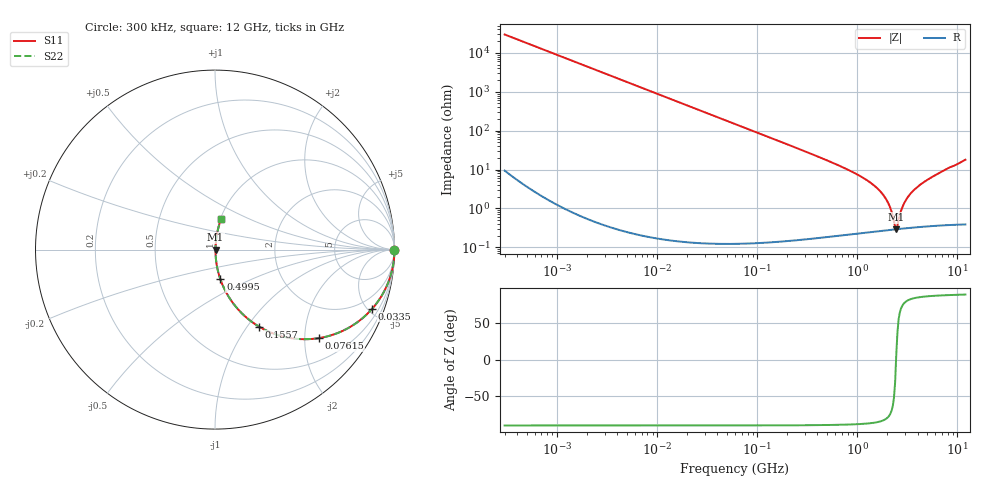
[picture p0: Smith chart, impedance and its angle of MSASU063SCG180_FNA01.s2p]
! MSASU063SCG180_FNA01  S-PARAMETER MODEL  ( Standard Model )
! Model Generated by TAIYO YUDEN Corporation (http://www.ty-top.com)
! Version 1.0
! TAIYO YUDEN Control No. 240819
! Copyright(c) 2024 TAIYO YUDEN CO.,LTD. All Rights Reserved.
! Product Description (link to TY-COMPAS)
! https://ds.yuden.co.jp/TYCOMPAS/or/detail?pn=MSASU063SCG180JFNA01&u=M
! Products Name : Multilayer Ceramic Capacitors
! Characteristics :
!  Capacitance : 18 [pF] , Rated Voltage : 50 [V] , TCC : CG / C0G
!  Case Size : 0.6 x 0.3 / 0.024 x 0.012 [mm/inch] , Thickness : 0.3 / 0.012 [mm/inch]
!  (Conditions: Temperature = 25 [degC] , DC Bias Voltage = 0 [V])
! External Node Assignments :
!  1  o---| |---o  2
! GND o---------o GND
! Frequency Range : 0.3MHz  -  12000MHz  [ 401 STEP ]
# MHZ S RI R 50
! Freq[MHz].  S11 Real  S11 Imag  S21 Real  S21 Imag  S12 Real  S12 Imag  S22 Real  S22 Imag
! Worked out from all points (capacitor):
!   401 points, 300 kHz to 12 GHz, reference 50 ohm
!   read as one part in series: C = 17.8 pF near 316.3 kHz
!   lowest |Z| = 293 mohm at 2.448 GHz (marker M1)
!   series resonance near 2.438 GHz, so ESL is about 240 pH
!   S11 on the Smith chart (normalised r, x): 300 kHz: open; 33.5 MHz: 1.00, -5.33; 76.15 MHz: 1.00, -2.34; 155.7 MHz: 1.00, -1.14; 499.5 MHz: 1.00, -0.34; 12 GHz: 1.01, +0.36
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0.3  1 -0.00336  1.24e-05 0.00336  1.24e-05 0.00336  1 -0.00336
1.769972  0.9996 -0.0198  0.000396 0.0198  0.000396 0.0198  0.9996 -0.0198
10.44266  0.9865 -0.1155  0.0135 0.1155  0.0135 0.1155  0.9865 -0.1155
33.49947  0.8763 -0.329  0.1237 0.329  0.1237 0.329  0.8763 -0.329
60  0.6882 -0.4628  0.3118 0.4628  0.3118 0.4628  0.6882 -0.4628
76.15486  0.578 -0.4934  0.422 0.4934  0.422 0.4934  0.578 -0.4934
107.4644  0.4072 -0.4905  0.5928 0.4905  0.5928 0.4905  0.4072 -0.4905
155.7172  0.2462 -0.4296  0.7538 0.4296  0.7538 0.4296  0.2462 -0.4296
353.9943  0.0588 -0.2319  0.9412 0.2319  0.9412 0.2319  0.0588 -0.2319
499.5319  0.0301 -0.1657  0.9699 0.1657  0.9699 0.1657  0.0301 -0.1657
918.7169  0.00904 -0.0824  0.991 0.0824  0.991 0.0824  0.00904 -0.0824
1366.97  0.00445 -0.0445  0.9955 0.0445  0.9955 0.0445  0.00445 -0.0445
1781.601  0.0032 -0.0233  0.9968 0.0233  0.9968 0.0233  0.0032 -0.0233
2088.533  0.00291 -0.0114  0.9971 0.0114  0.9971 0.0114  0.00291 -0.0114
2321.999  0.00287 -0.00367  0.9971 0.00367  0.9971 0.00367  0.00287 -0.00367
2448.343  0.0029 0.000347  0.9971 -0.000347  0.9971 -0.000347  0.0029 0.000347
2514.07  0.00293 0.00216  0.9971 -0.00216  0.9971 -0.00216  0.00293 0.00216
2795.104  0.0031 0.00967  0.9969 -0.00967  0.9969 -0.00967  0.0031 0.00967
3026.31  0.0033 0.0153  0.9967 -0.0153  0.9967 -0.0153  0.0033 0.0153
3740.715  0.00415 0.0305  0.9958 -0.0305  0.9958 -0.0305  0.00415 0.0305
5868.704  0.00823 0.0683  0.9918 -0.0683  0.9918 -0.0683  0.00823 0.0683
12000  0.0345 0.1719  0.9655 -0.1719  0.9655 -0.1719  0.0345 0.1719
